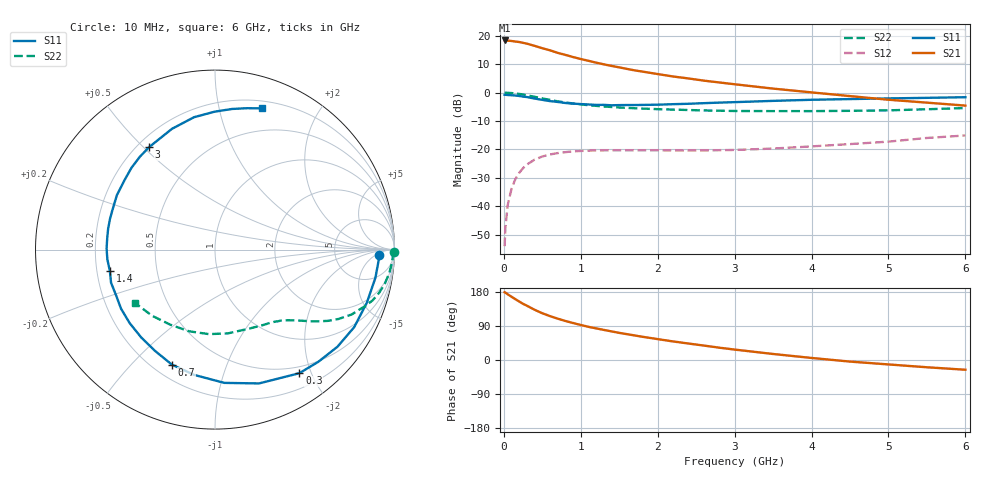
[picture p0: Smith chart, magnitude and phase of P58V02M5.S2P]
! SIEMENS Small Signal Semiconductors
! BFP183
! Si NPN RF Bipolar Junction Transistor in SOT143
! VCE = 8 V  IC = 2.5 mA
! Common Emitter S-Parameters:  March  1996
# GHz  S  MA  R  50
!  f  S11  S21  S12  S22
! GHz  MAG  ANG  MAG  ANG  MAG  ANG  MAG  ANG
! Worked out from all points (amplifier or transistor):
!   36 points, 10 MHz to 6 GHz, reference 50 ohm
!   highest |S21| = 18.3 dB at 10 MHz (marker M1)
!   |S21| within 3 dB of that: start of sweep to 536.2 MHz
!   unconditionally stable (mu >= 1): 2.057 GHz to 5.838 GHz
!   at 250 MHz: K = 0.14, MSG = 22.0 dB, |S12| = -26.6 dB
!   at 1.4 GHz: K = 0.72, MSG = 14.8 dB, |S12| = -20.3 dB
!   at 6 GHz: K = 0.97, MSG = 5.2 dB, |S12| = -15.1 dB
!   S11 on the Smith chart (normalised r, x): 10 MHz: 20, -7; 300 MHz: 0.40, -1.82; 700 MHz: 0.27, -0.66; 1.4 GHz: 0.25, -0.09; 3 GHz: 0.25, +0.52; 6 GHz: 0.27, +1.35
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0.01  0.9153 -1.9  8.233 178.8  0.002 85.7  0.9969 -0.7
0.02  0.9136 -3.9  8.17 177.9  0.0042 83.4  0.9917 -1.5
0.05  0.9074 -10.0  8.16 173.4  0.0105 84.9  0.9898 -3.7
0.1  0.8963 -19.3  8.062 166.9  0.0205 77.6  0.9802 -7.6
0.2  0.8709 -38.4  7.734 154.2  0.0389 68.7  0.9466 -14.6
0.25  0.8499 -47.3  7.48 148.2  0.047 63.9  0.9221 -17.9
0.3  0.8337 -55.7  7.227 143.2  0.0544 59.7  0.8938 -20.6
0.4  0.7849 -71.8  6.615 132.5  0.0663 51.7  0.8428 -25.4
0.5  0.7444 -86.0  6.01 123.4  0.0752 45.1  0.7896 -29.3
0.6  0.7076 -99.4  5.522 115.8  0.0817 39.7  0.7431 -32.3
0.7  0.6845 -110.5  4.982 109.1  0.0864 35.2  0.7016 -34.7
0.8  0.6557 -120.7  4.59 103.0  0.0897 31.6  0.6697 -36.6
0.9  0.6392 -130.0  4.21 97.6  0.0928 28.5  0.6431 -38.2
1.1  0.6183 -147.9  3.617 87.5  0.0955 23.5  0.5997 -41.1
1.4  0.5977 -168.5  2.939 75.5  0.0969 18.8  0.558 -44.9
1.8  0.6067 168.9  2.338 61.3  0.0967 16.2  0.5228 -50.1
2.2  0.6251 151.0  1.917 49.0  0.0961 15.3  0.502 -56.1
3  0.6788 122.7  1.399 27.5  0.0981 18.5  0.4744 -70.7
3.5  0.7144 109.6  1.174 15.9  0.1038 21.2  0.4724 -81.3
4.5  0.7686 90.1  0.867 -4.2  0.1244 24.3  0.4776 -107.7
5.5  0.8079 77.2  0.665 -19.2  0.1593 23.6  0.509 -133.7
6  0.8287 71.7  0.59 -25.7  0.1763 20.4  0.5347 -146.1
